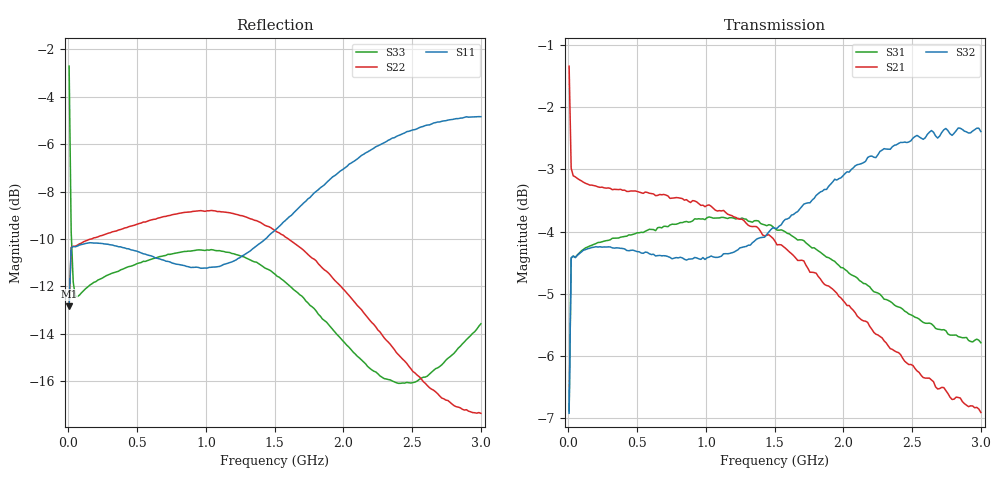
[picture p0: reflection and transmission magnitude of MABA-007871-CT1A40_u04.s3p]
#	MHz	S	RI	R	50
!FREQ	R1	I1	R2	I2	R3	I3
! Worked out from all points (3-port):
!   201 points, 5 MHz to 3 GHz, reference 50 ohm
!   strongest paths, dB at 5 MHz, 753.8 MHz, 1.502 GHz, 2.251 GHz, 3 GHz:
!     S32: -6.9, -4.4, -3.9, -2.8, -2.4
!     S21: -1.3, -3.5, -4.2, -5.7, -6.9
!     S31: -6.9, -3.9, -4.0, -5.0, -5.8
!   lowest |S11| = -12.8 dB at 5 MHz (marker M1), VSWR 1.59, Z = 65.1 + j22 ohm
!   |S11| at or under -10 dB: start of sweep to 1.433 GHz
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5  0.1619 0.1602  0.8395 -0.1664  -0.3242 -0.3163
   0.8405 -0.1662  0.1591 0.162  0.3214 0.318
   -0.3242 -0.3163  0.3163 0.3214  -0.3557 0.6398
19.975  0.2973 0.059  0.7041 -0.0835  -0.5879 -0.1229
        0.7044 -0.0842  0.2959 0.0685  0.586 0.1327
        -0.5879 -0.1229  0.5868 0.1317  0.1786 0.2743
34.95  0.304 0.0207  0.6965 -0.0648  -0.6011 -0.051
       0.6965 -0.0654  0.3029 0.0375  0.5996 0.0677
       -0.6011 -0.051  0.5991 0.0676  0.2061 0.1526
379.375  0.2457 -0.1797  0.6224 -0.2812  -0.5782 0.2361
         0.6219 -0.2808  0.3308 -0.0149  0.6103 -0.0462
         -0.5782 0.2361  0.61 -0.047  0.2704 0.0303
813.65  0.00937 -0.2788  0.4115 -0.5331  -0.4088 0.4945
        0.4141 -0.5283  0.3474 -0.0883  0.5937 -0.0988
        -0.4088 0.4945  0.5934 -0.1001  0.2961 -0.0157
1502.5  -0.3277 0.0365  -0.1178 -0.6003  0.0682 0.6309
        -0.1057 -0.6109  0.2467 -0.2185  0.6172 -0.1648
        0.0682 0.6309  0.6129 -0.1657  0.2454 -0.1038
1831.95  -0.2845 0.2889  -0.3208 -0.463  0.2724 0.5429
         -0.3194 -0.4821  0.1651 -0.2231  0.6435 -0.2342
         0.2724 0.5429  0.639 -0.2295  0.1921 -0.1019
2236.275  -0.0523 0.4923  -0.442 -0.2321  0.4225 0.3735
          -0.4609 -0.2451  0.0973 -0.1818  0.644 -0.3522
          0.4225 0.3735  0.6367 -0.3437  0.1549 -0.0589
2595.675  0.2061 0.5084  -0.4582 -0.0352  0.4846 0.2213
          -0.4803 -0.0302  0.0769 -0.1367  0.6016 -0.4699
          0.4846 0.2213  0.5972 -0.4547  0.1612 -0.0124
3000  0.4361 0.3712  -0.4085 0.1602  0.5107 0.0563
      -0.4137 0.1813  0.0846 -0.1059  0.4988 -0.588
      0.5107 0.0563  0.4969 -0.574  0.2086 0.0185
